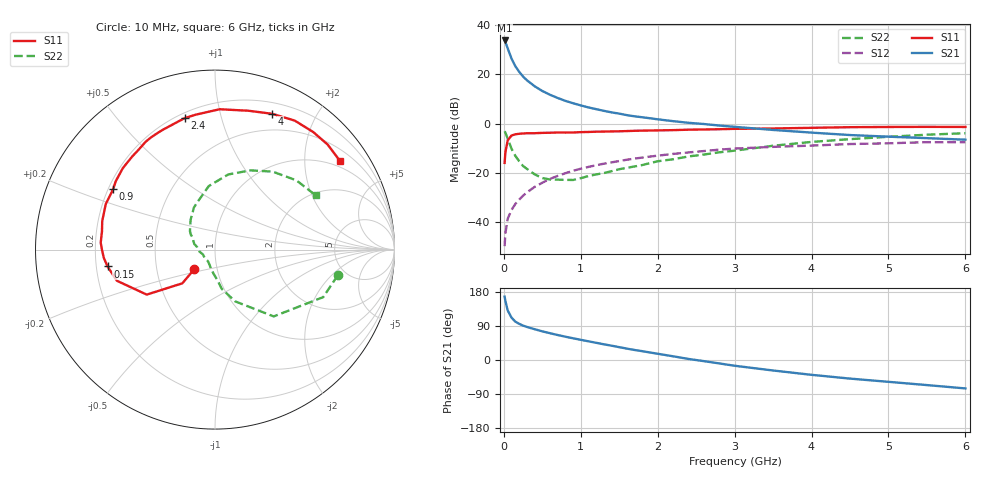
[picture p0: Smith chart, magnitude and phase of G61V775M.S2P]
! SIEMENS Small Signal Semiconductors
! BFG193
! Si NPN RF Bipolar Junction Transistor in SOT223
! VCE = 1.75 V  IC = 75 mA
! Common Emitter S-Parameters:  August  1996
# GHz  S  MA  R  50
!  f  S11  S21  S12  S22
! GHz  MAG  ANG  MAG  ANG  MAG  ANG  MAG  ANG
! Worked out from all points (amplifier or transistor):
!   36 points, 10 MHz to 6 GHz, reference 50 ohm
!   highest |S21| = 33.6 dB at 10 MHz (marker M1)
!   |S21| within 3 dB of that: start of sweep to 47.54 MHz
!   unconditionally stable (mu >= 1): start of sweep to 18.76 MHz; 168.8 MHz to 4.324 GHz; 5.527 GHz to end of sweep
!   at 250 MHz: K = 1.08, MAG = 22.4 dB, |S12| = -29.2 dB
!   at 1.4 GHz: K = 1.13, MAG = 7.9 dB, |S12| = -15.7 dB
!   at 6 GHz: K = 1.03, MAG = -0.5 dB, |S12| = -7.5 dB
!   S11 on the Smith chart (normalised r, x): 10 MHz: 0.77, -0.18; 150 MHz: 0.25, -0.07; 900 MHz: 0.22, +0.26; 2.4 GHz: 0.23, +0.77; 4 GHz: 0.31, +1.46; 6 GHz: 0.81, +2.95
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0.01  0.1599 -136.5  48.12 167.3  0.0033 71.7  0.699 -11.8
0.02  0.2616 -134.1  44.93 155.9  0.006 68.1  0.6585 -23.7
0.05  0.4556 -146.6  33.24 130.9  0.0118 62.5  0.4956 -48.7
0.1  0.5738 -162.4  20.63 111.7  0.0178 63.0  0.3091 -68.8
0.15  0.6061 -171.1  14.45 101.2  0.0237 63.3  0.2213 -80.3
0.2  0.6214 -175.8  11.12 95.4  0.0289 66.6  0.172 -85.2
0.25  0.6299 -180.0  8.955 90.7  0.0347 67.5  0.1382 -92.5
0.3  0.6379 176.5  7.529 87.2  0.0405 68.6  0.1213 -97.4
0.4  0.6379 170.8  5.702 81.3  0.0521 68.4  0.094 -107.8
0.5  0.6481 165.8  4.567 75.6  0.0634 67.3  0.0789 -117.5
0.6  0.6523 161.3  3.83 70.7  0.0758 66.4  0.0738 -126.7
0.7  0.6594 157.4  3.295 65.9  0.0873 64.9  0.0733 -137.6
0.9  0.6597 149.3  2.579 57.3  0.1107 61.0  0.0722 -158.0
1.1  0.6764 142.3  2.122 49.3  0.1325 56.8  0.0867 -172.4
1.6  0.7051 125.6  1.48 30.0  0.1856 45.1  0.1273 159.7
2.2  0.7365 108.4  1.119 9.8  0.243 30.5  0.1896 137.0
2.4  0.7518 103.0  1.037 2.8  0.2604 26.1  0.2161 128.9
3.5  0.7957 76.5  0.743 -27.7  0.3377 -2.3  0.3555 95.6
4  0.8208 67.2  0.656 -39.1  0.3582 -12.2  0.4252 80.0
4.5  0.8449 58.3  0.586 -49.1  0.3852 -22.5  0.484 65.8
5.5  0.8581 43.0  0.507 -66.2  0.4205 -45.6  0.5954 40.4
6  0.8539 35.2  0.472 -75.0  0.4197 -58.6  0.6379 28.2
